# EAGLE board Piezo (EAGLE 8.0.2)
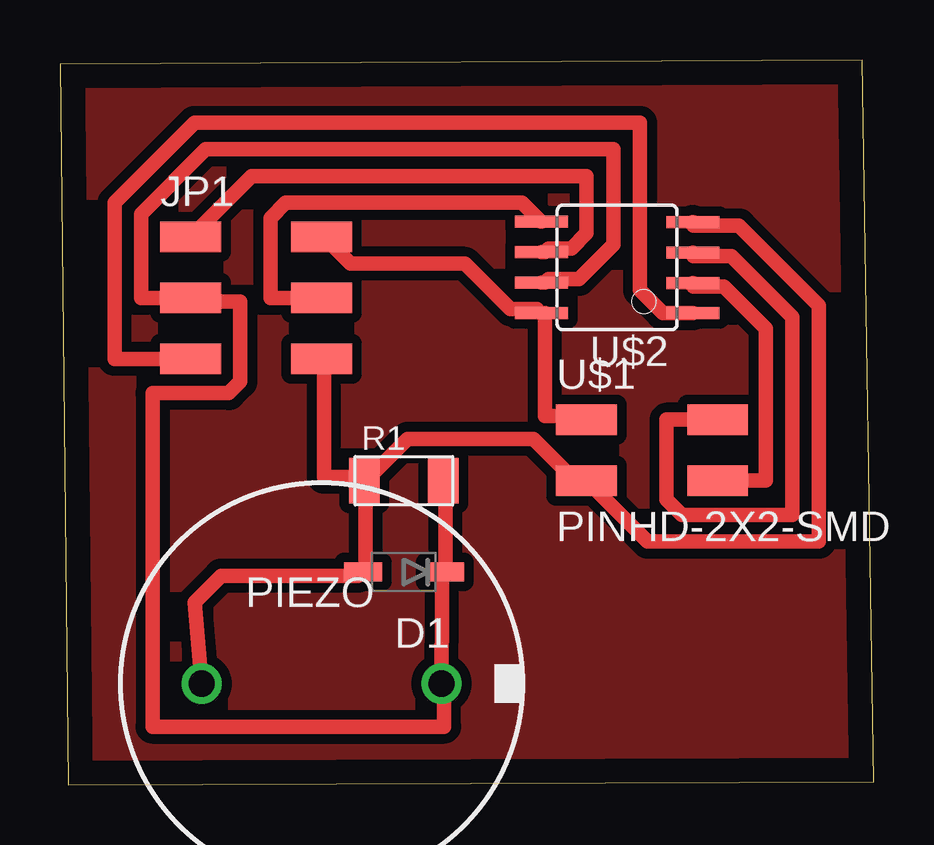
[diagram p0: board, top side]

Size 33.92 x 30.22 mm. Coordinates in mm from the lower left corner, seen from the top.
Outline: 0.35,0 33.92,0.12 33.45,30.22 0,30.05 0.35,0
Copper layers (1*16): Top 0.035mm / dielectric 1.5mm / Bottom 0.035mm
Design rules "default *": minimum track width 24mil, minimum drill 24mil, track to track 16mil, track to pad 16mil, pad to pad 16mil, via to via 16mil, smd to smd 8mil, copper to edge 40mil, drill to drill 8mil, minimum pad ring 10mil, minimum via ring 8mil, stop-mask expansion 4mil, vias tented up to drill 0mil, thermal gap 10mil

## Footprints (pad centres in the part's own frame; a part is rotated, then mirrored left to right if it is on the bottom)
SOD123 = smd 1.6 x 0.8: ANODE 1.7,0; CATHODE -1.7,0
2X03SMD = smd 2.54 x 1.27: 1 -2.54,2.54; 2 2.92,2.54; 3 -2.54,0; 4 2.92,0; 5 -2.54,-2.54; 6 2.92,-2.54
EFBAA40D101 = drill 1.1 pad 1.676: 1 -5,0; 2 5,0
R1206FAB = smd 1.27 x 1.905: 1 -1.651,0; 2 1.651,0
2X02SMD = smd 2.54 x 1.27: 1 -2.54,1.27; 2 2.92,1.27; 3 -2.54,-1.27; 4 2.92,-1.27
SOIC8 = smd 0.5 x 2.2: 1 -1.905,-3.154; 2 -0.645,-3.154; 3 0.625,-3.154; 4 1.895,-3.154; 5 1.905,3.154; 6 0.635,3.154; 7 -0.635,3.154; 8 -1.905,3.154

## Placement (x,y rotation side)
D1  4.7  [SOD123]  14.34,8.87 180 top
JP1  [2X03SMD]  7.99,20.3 0 top
PIEZO  EFBAA40D101  [EFBAA40D101]  10.91,4.22 0 top
R1  1M  [R1206FAB]  14.34,12.68 0 top
U$1  PINHD-2X2-SMD  [2X02SMD]  24.5,13.95 0 top
U$2  ATTINY45SI  [SOIC8]  23.23,21.57 90 top

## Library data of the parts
D1 R1 U$1 = fab
JP1 = 01_FAB_Hello
PIEZO = buzzer; OC_FARNELL: unknown; OC_NEWARK: unknown
U$2 = 01_fab

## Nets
GND: D1.ANODE JP1.6 PIEZO.1 R1.1 U$1.3 U$2.4
MISO: JP1.1 U$2.6
MOSI: JP1.4 U$2.5
RST: JP1.5 U$2.1
RX: U$1.4 U$2.2
SCK: D1.CATHODE JP1.3 PIEZO.2 R1.2 U$2.7
TX: U$1.2 U$2.3
VCC: JP1.2 U$1.1 U$2.8

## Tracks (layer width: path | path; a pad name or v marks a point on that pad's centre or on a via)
GND
  Top 0.61: R1.1 12.75,12.68 12.75,8.87 D1.ANODE 12.43,8.71 6.72,8.71 5.61,7.6 PIEZO.1 | JP1.6 11,17.76 11,12.84 12.43,12.84 R1.1 | U$2.4 26.4,23.32 28.31,23.32 31.64,19.99 31.64,10.14 24.5,10.14 U$1.3 21.8,12.84 21.32,12.84 19.73,14.43 14.5,14.43 12.91,12.84 R1.1
MISO
  Top 0.61: JP1.1 7.99,25.38 21.96,25.38 21.96,23 21.32,22.37 20.37,22.37 20.21,22.21 U$2.6
MOSI
  Top 0.61: JP1.4 8.78,20.3 8.78,23.64 9.42,24.27 19.26,24.27 20.05,23.48 U$2.5
N$1
  pour Top: 1.71,29.78 0.4,29.78 0.84,0.36 33.64,0.38 33.19,29.71
RST
  Top 0.61: U$2.1 25.13,19.67 24.18,20.62 24.18,27.61 5.61,27.61 2.27,24.27 2.27,17.76 JP1.5
RX
  Top 0.61: U$1.4 29.42,12.68 29.42,19.03 27.67,20.78 26.4,20.78 U$2.2
SCK
  Top 0.61: R1.2 16.08,12.68 16.08,9.03 D1.CATHODE 15.92,8.87 15.92,7.6 PIEZO.2 16.02,4.22 16.02,2.43 3.86,2.43 3.86,16.33 7.03,16.33 7.51,16.81 7.51,20.14 5.61,20.14 JP1.3 3.38,20.3 3.38,23.8 6.08,26.49 23.07,26.49 23.07,22.53 21.64,21.1 20.37,21.1 20.21,20.94 U$2.7
TX
  Top 0.61: U$1.2 25.29,15.22 25.29,11.89 25.93,11.25 30.53,11.25 30.53,19.51 27.99,22.05 26.4,22.05 U$2.3
VCC
  Top 0.61: U$1.1 21.8,15.38 20.21,15.38 20.21,19.67 U$2.8 19.89,19.83 18.78,19.83 16.88,21.73 12.12,21.73 11,22.84 JP1.2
